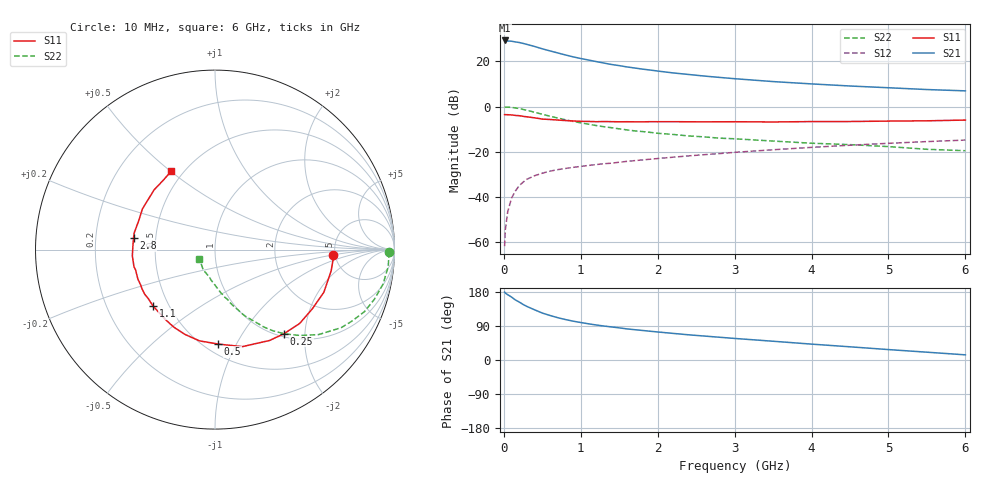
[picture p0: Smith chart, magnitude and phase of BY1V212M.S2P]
! SIEMENS Small Signal Semiconductors
! BFY420
! Si NPN RF SIEGET Grounded Emitter Transistor in MICRO-X
! VCE = 1.25 V  IC = 12 mA
! Common Emitter S-Parameters:  October  1996
# GHz  S  MA  R  50
!  f  S11  S21  S12  S22
! GHz  MAG  ANG  MAG  ANG  MAG  ANG  MAG  ANG
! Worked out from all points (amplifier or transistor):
!   36 points, 10 MHz to 6 GHz, reference 50 ohm
!   highest |S21| = 29.3 dB at 10 MHz (marker M1)
!   |S21| within 3 dB of that: start of sweep to 431.7 MHz
!   unconditionally stable (mu >= 1): 2.278 GHz to end of sweep
!   at 250 MHz: K = 0.22, MSG = 30.8 dB, |S12| = -33.6 dB
!   at 1.4 GHz: K = 0.82, MSG = 21.9 dB, |S12| = -25.1 dB
!   at 6 GHz: K = 1.10, MAG = 9.0 dB, |S12| = -14.9 dB
!   S11 on the Smith chart (normalised r, x): 10 MHz: 4.82, -0.49; 250 MHz: 1.06, -1.57; 500 MHz: 0.58, -0.85; 1.1 GHz: 0.41, -0.33; 2.8 GHz: 0.37, +0.06; 6 GHz: 0.43, +0.50
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0.01  0.6597 -2.5  29.19 179.2  0.0008 92.6  0.9697 -0.8
0.02  0.6604 -4.9  29.12 176.5  0.0019 81.5  0.9696 -2.1
0.1  0.6514 -21.4  28.06 166.1  0.0093 82.6  0.9556 -11.7
0.15  0.6347 -31.4  27.1 158.5  0.0134 75.3  0.9301 -17.3
0.2  0.6259 -41.1  26.28 153.0  0.0176 72.6  0.9019 -22.5
0.25  0.6063 -50.6  25.12 146.6  0.021 67.6  0.8614 -27.5
0.3  0.5906 -59.0  23.86 141.3  0.0244 66.0  0.8263 -31.8
0.4  0.5617 -74.3  21.46 132.4  0.0292 60.3  0.7462 -39.4
0.5  0.5266 -88.0  19.04 123.9  0.0332 56.1  0.6731 -45.3
0.6  0.5158 -99.6  17.12 117.5  0.0369 53.5  0.6094 -50.4
0.7  0.5014 -109.5  15.45 111.7  0.0398 51.9  0.5556 -54.5
0.8  0.4891 -118.0  13.93 106.8  0.0423 49.9  0.5079 -57.9
0.9  0.478 -125.0  12.64 102.5  0.0448 49.5  0.4676 -60.4
1.1  0.4666 -137.9  10.76 95.5  0.0494 49.0  0.4056 -65.7
1.3  0.4638 -147.5  9.215 89.7  0.0539 48.3  0.3568 -69.3
1.6  0.46 -158.9  7.555 82.1  0.0608 48.1  0.3031 -74.5
2.2  0.4617 -175.9  5.564 70.2  0.0752 47.1  0.2405 -82.6
2.8  0.4586 171.9  4.429 60.1  0.0904 45.2  0.199 -89.7
3.5  0.4544 159.3  3.574 49.5  0.11 41.6  0.1715 -97.2
4.5  0.4652 143.3  2.852 34.8  0.1386 34.5  0.1428 -109.3
5.5  0.4821 126.7  2.38 20.6  0.1668 25.9  0.1126 -132.3
6  0.501 119.0  2.226 13.6  0.1802 21.1  0.1047 -148.4
